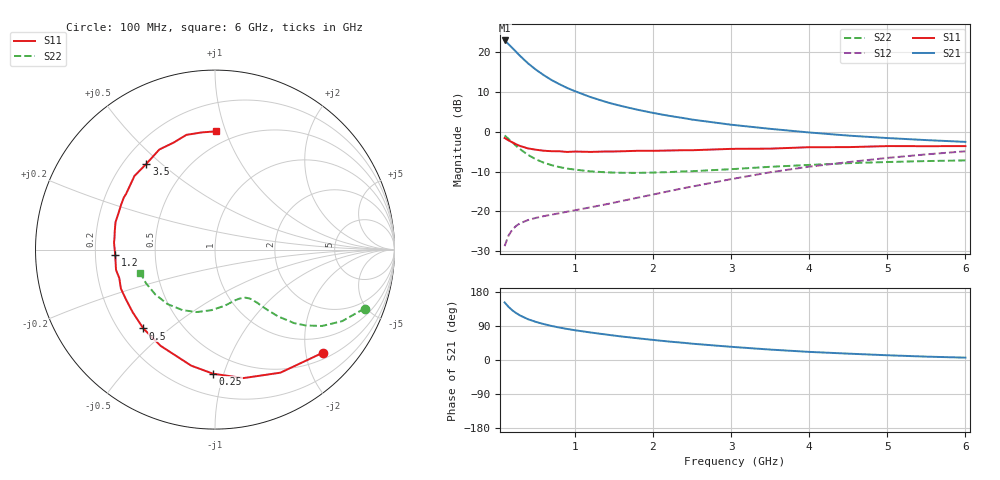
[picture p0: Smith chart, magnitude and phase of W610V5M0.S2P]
! SIEMENS Small Signal Semiconductors
! BFR193W
! Si NPN RF Bipolar Junction Transistor in SOT323
! VCE = 10 V  IC = 5 mA
! Common Emitter S-Parameters:  September  1992
# GHz  S  MA  R  50
!  f  S11  S21  S12  S22
! GHz  MAG  ANG  MAG  ANG  MAG  ANG  MAG  ANG
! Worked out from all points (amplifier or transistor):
!   28 points, 100 MHz to 6 GHz, reference 50 ohm
!   highest |S21| = 22.8 dB at 100 MHz (marker M1)
!   |S21| within 3 dB of that: start of sweep to 254.3 MHz
!   unconditionally stable (mu >= 1): 1.234 GHz to 2.608 GHz
!   at 300 MHz: K = 0.35, MSG = 20.9 dB, |S12| = -23.0 dB
!   at 1.5 GHz: K = 1.06, MAG = 10.9 dB, |S12| = -17.8 dB
!   at 6 GHz: K = 0.88, MSG = 1.2 dB, |S12| = -4.9 dB
!   S11 on the Smith chart (normalised r, x): 100 MHz: 0.63, -2.36; 250 MHz: 0.35, -0.92; 500 MHz: 0.30, -0.41; 1.2 GHz: 0.28, -0.02; 3.5 GHz: 0.29, +0.45; 6 GHz: 0.40, +0.92
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0.1  0.8319 -43.6  13.88 151.9  0.0367 67.8  0.8955 -21.5
0.15  0.7766 -62.0  12.5 140.3  0.0499 59.7  0.8125 -29.4
0.2  0.7332 -77.5  11.16 130.9  0.0592 53.7  0.7327 -35.5
0.25  0.6916 -90.9  9.924 123.5  0.0662 49.2  0.6589 -39.9
0.3  0.66 -101.6  8.848 117.3  0.0712 46.5  0.6017 -42.9
0.4  0.6159 -119.5  7.17 107.6  0.078 42.8  0.5106 -46.7
0.5  0.5936 -132.3  5.98 100.6  0.083 41.8  0.4505 -48.8
0.6  0.5764 -142.7  5.113 94.9  0.0872 41.7  0.4085 -50.4
0.7  0.5684 -150.7  4.436 89.9  0.0911 42.6  0.3805 -51.4
0.8  0.5676 -157.5  3.94 85.7  0.0948 43.8  0.36 -52.7
0.9  0.5564 -163.3  3.529 82.0  0.0992 45.4  0.3444 -53.4
1  0.5629 -168.4  3.214 78.6  0.1033 46.9  0.3343 -54.7
1.2  0.5569 -177.0  2.71 72.6  0.1126 50.0  0.3176 -57.5
1.4  0.5639 176.1  2.351 67.2  0.1229 53.1  0.3093 -60.6
1.6  0.5673 170.1  2.089 62.0  0.1351 55.8  0.3049 -64.1
1.8  0.575 164.6  1.882 57.4  0.1484 58.1  0.304 -68.1
2.2  0.5799 154.4  1.581 48.8  0.179 61.2  0.311 -76.0
3  0.608 137.6  1.221 34.8  0.2539 62.4  0.3383 -93.5
3.5  0.612 128.7  1.084 27.5  0.3095 60.2  0.3624 -106.2
4.5  0.6394 111.0  0.892 16.8  0.4148 52.4  0.4026 -131.1
5.5  0.6571 96.3  0.783 8.9  0.5188 42.9  0.4276 -154.0
6  0.6585 89.7  0.744 6.2  0.567 37.3  0.4358 -162.9
